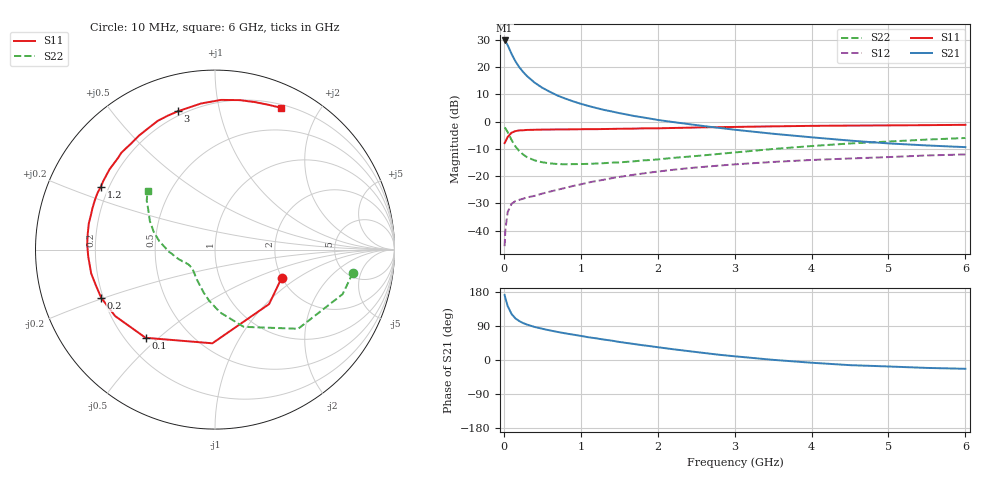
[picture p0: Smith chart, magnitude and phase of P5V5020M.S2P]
! SIEMENS Small Signal Semiconductors
! BFP183
! Si NPN RF Bipolar Junction Transistor in SOT143
! VCE = 0.5 V  IC = 20 mA
! Common Emitter S-Parameters:  March  1996
# GHz  S  MA  R  50
!  f  S11  S21  S12  S22
! GHz  MAG  ANG  MAG  ANG  MAG  ANG  MAG  ANG
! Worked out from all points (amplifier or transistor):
!   36 points, 10 MHz to 6 GHz, reference 50 ohm
!   highest |S21| = 29.7 dB at 10 MHz (marker M1)
!   |S21| within 3 dB of that: start of sweep to 69.85 MHz
!   unconditionally stable (mu >= 1): start of sweep to 10.37 MHz; 345.4 MHz to end of sweep
!   at 250 MHz: K = 0.80, MSG = 23.3 dB, |S12| = -28.3 dB
!   at 1.4 GHz: K = 1.70, MAG = 7.4 dB, |S12| = -20.8 dB
!   at 6 GHz: K = 1.42, MAG = -2.5 dB, |S12| = -12.0 dB
!   S11 on the Smith chart (normalised r, x): 10 MHz: 1.99, -0.76; 100 MHz: 0.28, -0.45; 200 MHz: 0.19, -0.20; 1.2 GHz: 0.17, +0.25; 3 GHz: 0.18, +0.75; 6 GHz: 0.23, +1.55
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0.01  0.4034 -23.3  30.69 171.5  0.0052 80.2  0.7794 -9.6
0.02  0.4278 -45.2  29.97 163.4  0.0104 72.9  0.7527 -19.3
0.05  0.5222 -91.6  25.1 142.3  0.022 57.7  0.6396 -43.6
0.1  0.6253 -128.2  17.45 121.5  0.031 41.6  0.4592 -69.6
0.15  0.6685 -146.4  12.78 109.9  0.0349 35.8  0.3514 -85.3
0.2  0.6886 -157.0  9.965 102.7  0.0368 34.0  0.288 -96.3
0.25  0.6935 -163.7  8.138 97.5  0.0385 34.0  0.2499 -104.3
0.3  0.7026 -169.1  6.845 93.6  0.0407 35.2  0.2231 -110.9
0.4  0.7074 -176.9  5.176 87.2  0.0435 37.2  0.1944 -121.4
0.5  0.7127 177.6  4.163 82.4  0.0479 39.4  0.1794 -128.8
0.6  0.7146 172.6  3.506 78.0  0.052 41.7  0.1712 -134.0
0.7  0.7181 168.2  2.991 74.0  0.0564 43.6  0.1667 -138.1
0.9  0.7207 161.3  2.351 67.0  0.066 45.9  0.166 -144.3
1.1  0.7267 154.4  1.934 60.0  0.0765 46.8  0.1679 -149.0
1.2  0.7263 151.2  1.776 57.2  0.0811 46.7  0.17 -151.0
1.7  0.7437 136.4  1.261 42.0  0.1067 45.3  0.1872 -159.0
2.2  0.7632 123.8  0.98 28.4  0.1308 41.1  0.2161 -167.4
3  0.7978 105.1  0.709 9.8  0.1642 33.0  0.2715 179.1
3.5  0.8174 95.6  0.598 0.4  0.1821 27.9  0.3142 171.4
4.5  0.8443 80.5  0.448 -13.6  0.2106 17.6  0.397 156.2
5.5  0.86 69.7  0.365 -20.9  0.2394 8.8  0.4678 144.4
6  0.8719 64.9  0.34 -23.2  0.2498 3.9  0.4998 138.8
